PROGRAM FAST
VAR
   (* background communication with the EL6001 as Master device *)
   COMportControl_MASTER: SerialLineControl;
   COMportControlError_MASTER: BOOL;
   COMportControlErrorID_MASTER: ComError_t;
END_VAR

COMportControl_MASTER(
   Mode:= SERIALLINEMODE_EL6_22B,
   pComIn:= ADR(COMin_EL6001_MASTER),(* I/O data; see global variables *)
   pComOut:= ADR(COMout_EL6001_MASTER),(* I/O data; see global variables *)
   SizeComIn:= SIZEOF(COMin_EL6001_MASTER),(* I/O data; see global variables *)
   TxBuffer:= TxBuffer_MASTER,(* transmit buffer; see global variables *)
   RxBuffer:= RxBuffer_MASTER,(* receive buffer; see global variables *)
   Error=> COMportControlError_MASTER,(* indicating an error *)
   ErrorID=> COMportControlErrorID_MASTER );(* contains the error-ID *)

END_PROGRAM
